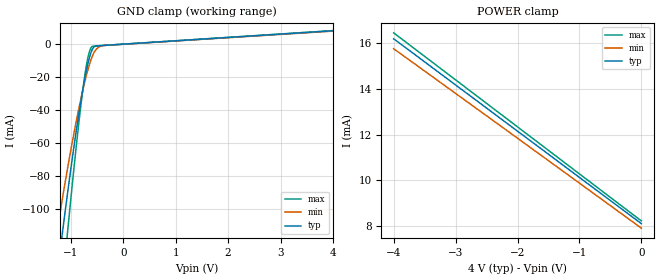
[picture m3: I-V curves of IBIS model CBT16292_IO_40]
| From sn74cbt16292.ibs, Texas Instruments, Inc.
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[Model]   CBT16292_IO_40
Model_type  Terminator
| variable   typ   min   max
C_comp   3.57pF   2.88pF   4.44pF
| C_tri-state   3.57pF   2.88pF   4.44pF
[Temperature Range]   40   100   -40
| Ambient temperature   25   85   -40
[Voltage range]   4   4   4
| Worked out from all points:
|   GND clamp passes 1 mA (typ) near -0.47 V on its own axis
[GND Clamp]
| CBT16292_IO_40
|   Voltage   I(typ)   I(min)   I(max)
-4V       -2.5A      -2.537A    -2.272A
-1.315V   -153.7mA   -123.8mA   -199.8mA
-1.225V   -130.2mA   -105.7mA   -168.2mA
-1.14V    -108.7mA   -89.31mA   -139.1mA
-1.055V   -88.08mA   -73.62mA   -110.9mA
-910mV    -55.09mA   -48.71mA   -65.45mA
-775mV    -27.95mA   -28.21mA   -28.15mA
-675mV    -11.71mA   -15.43mA   -7.971mA
-595mV    -3.34mA    -7.552mA   -1.364mA
-510mV    -1.124mA   -2.841mA   -1.053mA
-370mV    -752.1uA   -798uA     -761.8uA
4V        8.109mA    7.914mA    8.231mA
[POWER Clamp]
| CBT16292_IO_40
|   Voltage   I(typ)   I(min)   I(max)
-4V       16.19mA    15.76mA    16.45mA
-2.88V    13.93mA    13.57mA    14.15mA
-1.95V    12.05mA    11.75mA    12.24mA
-63.13fV  8.109mA    7.914mA    8.231mA
